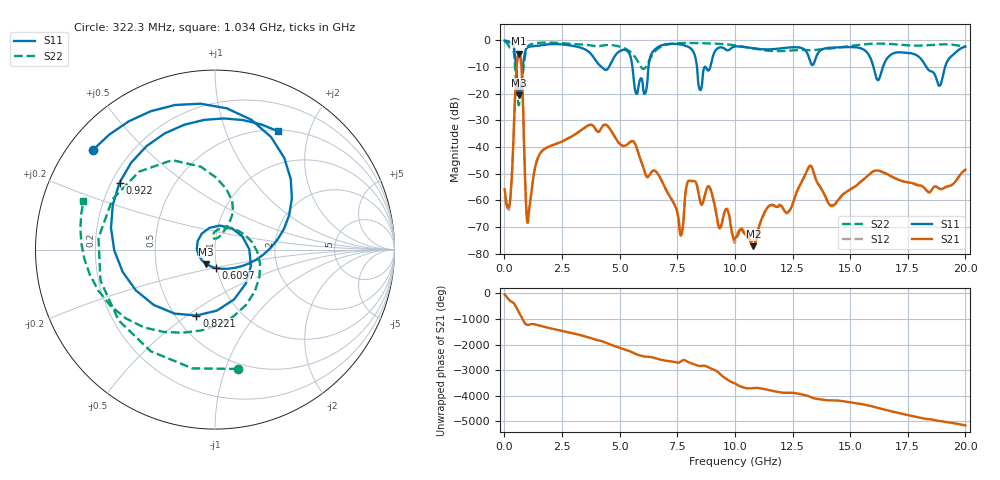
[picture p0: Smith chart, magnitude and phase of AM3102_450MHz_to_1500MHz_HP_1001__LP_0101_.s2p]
!Agilent Technologies,E8364B,MY43040894,A.07.50.67
!Agilent E8364B: A.07.50.67
!Date: Thursday, January 11, 2018 06:02:20
!Correction: S11(Full 2 Port(1,2))
!S21(Full 2 Port(1,2))
!S12(Full 2 Port(1,2))
!S22(Full 2 Port(1,2))
!S2P File: Measurements: S11, S21, S12, S22:
# Hz S  dB  R 50
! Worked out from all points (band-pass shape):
!   1601 points, 10 MHz to 20 GHz, reference 50 ohm
!   highest |S21| = -5.04 dB at 622.2 MHz (marker M1); lowest = -77.2 dB at 10.8 GHz (marker M2)
!   |S21| within 3 dB of the highest: 552.2 MHz to 724.5 MHz (172.3 MHz wide, 27 % of centre)
!   lowest |S11| = -20.6 dB at 634.7 MHz (marker M3), VSWR 1.21, Z = 44.8 - j7.26 ohm
!   |S11| at or under -10 dB: 5.555 GHz to 6.249 GHz (694.1 MHz wide, 11.8 % of centre); 16.01 GHz to 16.42 GHz (411.2 MHz wide, 2.54 % of centre); 18.3 GHz to 19.12 GHz (816.6 MHz wide, 4.36 % of centre)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
!   |S22| runs from -24.3 to -0.5 dB; largest |S21 - S12| = 0.0072
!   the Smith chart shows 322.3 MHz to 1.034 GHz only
!   S11 on the Smith chart (normalised r, x): 322.3 MHz: 0.07, +0.35; 609.7 MHz: 0.99, -0.21; 822.1 MHz: 0.63, -0.54; 922 MHz: 0.23, +0.30; 1.034 GHz: 0.51, +1.54
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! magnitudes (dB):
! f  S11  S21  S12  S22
! 10 MHz  -0.1  -55.8  -58.7  -0.5
! 322.3 MHz  -1.1  -51.0  -51.3  -3.4
! 609.7 MHz  -19.7  -5.2  -5.2  -24.0
! 622.2 MHz  -20.3  -5.0  -5.1  -24.3
! 634.7 MHz  -20.6  -5.0  -5.1  -24.2
! 822.1 MHz  -8.4  -28.3  -28.9  -10.7
! 922 MHz  -3.7  -57.7  -57.6  -4.6
! 1.034 GHz  -2.5  -67.4  -66.5  -2.1
! 1.559 GHz  -1.9  -42.3  -42.3  -0.9
! 3.346 GHz  -2.9  -33.6  -33.6  -1.6
! 6.094 GHz  -20.0  -49.6  -49.5  -10.5
! 6.682 GHz  -2.5  -50.4  -50.2  -3.0
! 7.669 GHz  -1.6  -73.1  -72.0  -1.0
! 7.981 GHz  -2.5  -52.8  -52.8  -1.0
! 8.493 GHz  -18.7  -60.4  -60.2  -1.1
! 10.01 GHz  -2.3  -74.1  -75.8  -1.9
! 10.8 GHz  -3.0  -77.2  -75.4  -3.1
! 13.34 GHz  -9.2  -47.6  -47.6  -3.8
! 14.2 GHz  -2.7  -62.1  -61.9  -3.0
! 16.68 GHz  -6.1  -50.5  -50.5  -1.3
! 18.88 GHz  -17.1  -55.6  -55.7  -1.5
! 20 GHz  -2.4  -48.5  -48.6  -2.3
